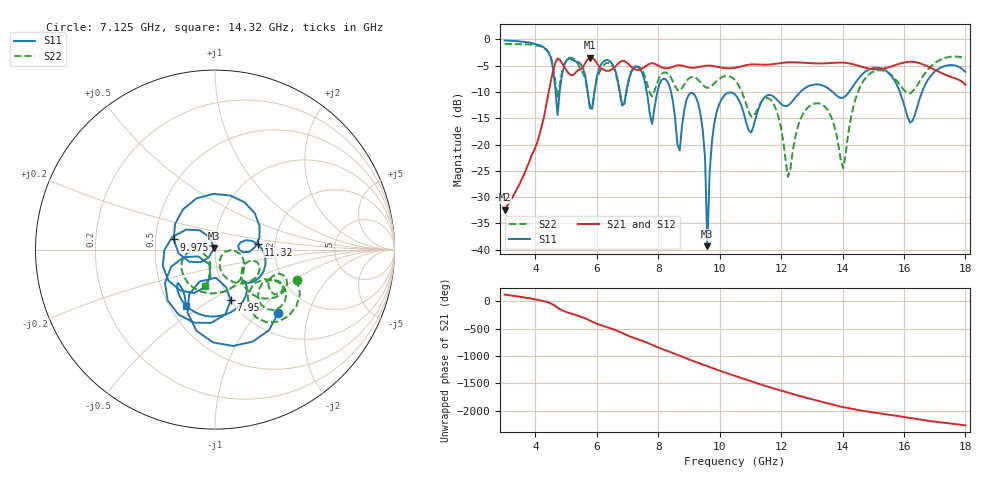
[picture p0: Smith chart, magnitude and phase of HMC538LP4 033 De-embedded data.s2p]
! Chelmsford, MA 01824
! http://www.hittite.com
! Tel: 978-250-3343
! Fax: 978-250-3373
! Device  :  HMC538LP4
! Description:  600 Analog Phase Shifter
! Frequency  :  6.0 GHz - 15.0 GHz
! Package  :  LP4  - 4x4 mm Quad Flatpack No-Lead (QFN) Plastic Package: 24 pin
! Ports  :  2 RF, 1 DC
!  Pin  3  = Rfin  = Port 1
!  Pin  16  = Rfout = Port 2
!  pin  21  = vCTL
! Voltages:  VCTL  = 0 to 5.0 Volts
! Currents :  Vb(V)  Vd(V)  Ib(mA)  Id(mA)
!  0.00  3.30  0.000000	0.476437
! Data:  The device was measured on evaluation board 111296-1.
!  Data was collected using a calibrated network analyzer.
!  The evaluation circuit board was modeled and simulated.This was use
!  to removed the evaluation board circuit from the measured data.
!  The reference plane is the center of the package pin.
! Misc:  Lot #
!Date Measured:  03 - 11 -2009
! Date:  03 - 17 -2009
! Note:
!  Hittite Microwave supplies this data as a sample of measured data at the
!  package pin for this package product.  Your particular data for this product
!  may vary.
!  Data was taken at 25 degrees C.
!  Hittite Microwave reserves the right to change this data at anytime.
# MHz S MA R 50
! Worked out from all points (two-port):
!   201 points, 3 GHz to 18 GHz, reference 50 ohm
!   highest |S21| = -3.49 dB at 5.775 GHz (marker M1); lowest = -32.4 dB at 3 GHz (marker M2)
!   |S21| within 3 dB of the highest: 4.557 GHz to 5.097 GHz (540.2 MHz wide, 11.2 % of centre); 5.279 GHz to 17.26 GHz (11.98 GHz wide, 106 % of centre)
!   lowest |S11| = -39.3 dB at 9.6 GHz (marker M3), VSWR 1.02, Z = 49.5 + j0.969 ohm
!   |S11| at or under -10 dB: 8.417 GHz to 12.63 GHz (4.211 GHz wide, 40 % of centre); 13.68 GHz to 14.21 GHz (529.9 MHz wide, 3.8 % of centre); 15.87 GHz to 16.59 GHz (724 MHz wide, 4.46 % of centre)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
!   |S22| runs from -26.2 to -0.8 dB; largest |S21 - S12| = 0.0037
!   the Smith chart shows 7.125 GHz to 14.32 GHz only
!   S11 on the Smith chart (normalised r, x): 7.125 GHz: 1.39, -1.30; 7.95 GHz: 1.00, -0.62; 9.975 GHz: 0.62, +0.07; 11.32 GHz: 1.63, +0.10; 14.32 GHz: 0.60, -0.43
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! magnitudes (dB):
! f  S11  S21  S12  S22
! 3 GHz  -0.2  -32.4  -32.4  -0.8
! 4.425 GHz  -2.5  -10.3  -10.3  -2.4
! 4.725 GHz  -14.4  -3.6  -3.7  -11.0
! 5.55 GHz  -5.4  -5.3  -5.3  -6.4
! 5.775 GHz  -13.1  -3.5  -3.5  -12.6
! 7.125 GHz  -6.1  -5.2  -5.2  -6.2
! 7.95 GHz  -10.6  -4.8  -4.8  -8.6
! 8.025 GHz  -8.7  -5.1  -5.1  -7.4
! 8.7 GHz  -21.1  -4.9  -4.9  -9.8
! 9.3 GHz  -12.1  -5.3  -5.3  -7.7
! 9.525 GHz  -22.5  -5.0  -5.0  -9.0
! 9.6 GHz  -39.3  -5.0  -5.0  -9.2
! 9.975 GHz  -12.5  -5.3  -5.3  -7.6
! 10.5 GHz  -10.5  -5.4  -5.4  -7.7
! 11.32 GHz  -12.3  -4.8  -4.8  -12.2
! 12.22 GHz  -12.6  -4.4  -4.4  -26.2
! 13.05 GHz  -8.6  -4.6  -4.6  -12.3
! 14.03 GHz  -11.1  -4.4  -4.4  -24.5
! 14.32 GHz  -9.1  -4.7  -4.7  -13.5
! 15.53 GHz  -6.5  -5.3  -5.3  -6.5
! 16.2 GHz  -15.8  -4.2  -4.3  -10.2
! 18 GHz  -6.2  -8.6  -8.6  -3.6
